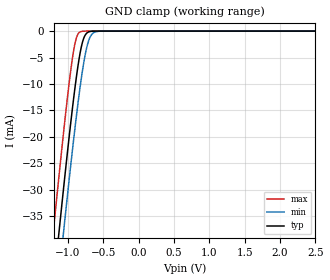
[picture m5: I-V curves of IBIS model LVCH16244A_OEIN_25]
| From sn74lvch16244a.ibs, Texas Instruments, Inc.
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[Model]   LVCH16244A_OEIN_25
Model_type  Input
Vinl=0.7
Vinh=1.7
| variable   typ   min   max
C_comp   3.49pF   2.69pF   4.69pF
[Temperature Range]   40   100   -40
| Ambient temperature   25   85   -40
[Voltage range]   2.5   2.3   2.7
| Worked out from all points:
|   GND clamp passes 1 mA (typ) near -0.77 V on its own axis
[GND Clamp]
| LVCH16244A_OEIN_25
|   Voltage   I(typ)   I(min)   I(max)
-5V       -583.8mA   -590.8mA   -575.1mA
-1.205V   -48.27mA   -56.56mA   -37.63mA
-1.13V    -38.42mA   -46.71mA   -27.77mA
-1.07V    -30.71mA   -38.96mA   -20.13mA
-1.05V    -28.19mA   -36.42mA   -17.65mA
-955mV    -16.68mA   -24.66mA   -6.874mA
-885mV    -9.098mA   -16.55mA   -1.486mA
-830mV    -4.281mA   -10.75mA   -171.6uA
-780mV    -1.472mA   -6.227mA   -17.15uA
-710mV    -173.7uA   -1.918mA   -639nA
-645mV    -18.49uA   -387.7uA   -29.98nA
2.5V      4.713pA    7.577pA    4.389pA
